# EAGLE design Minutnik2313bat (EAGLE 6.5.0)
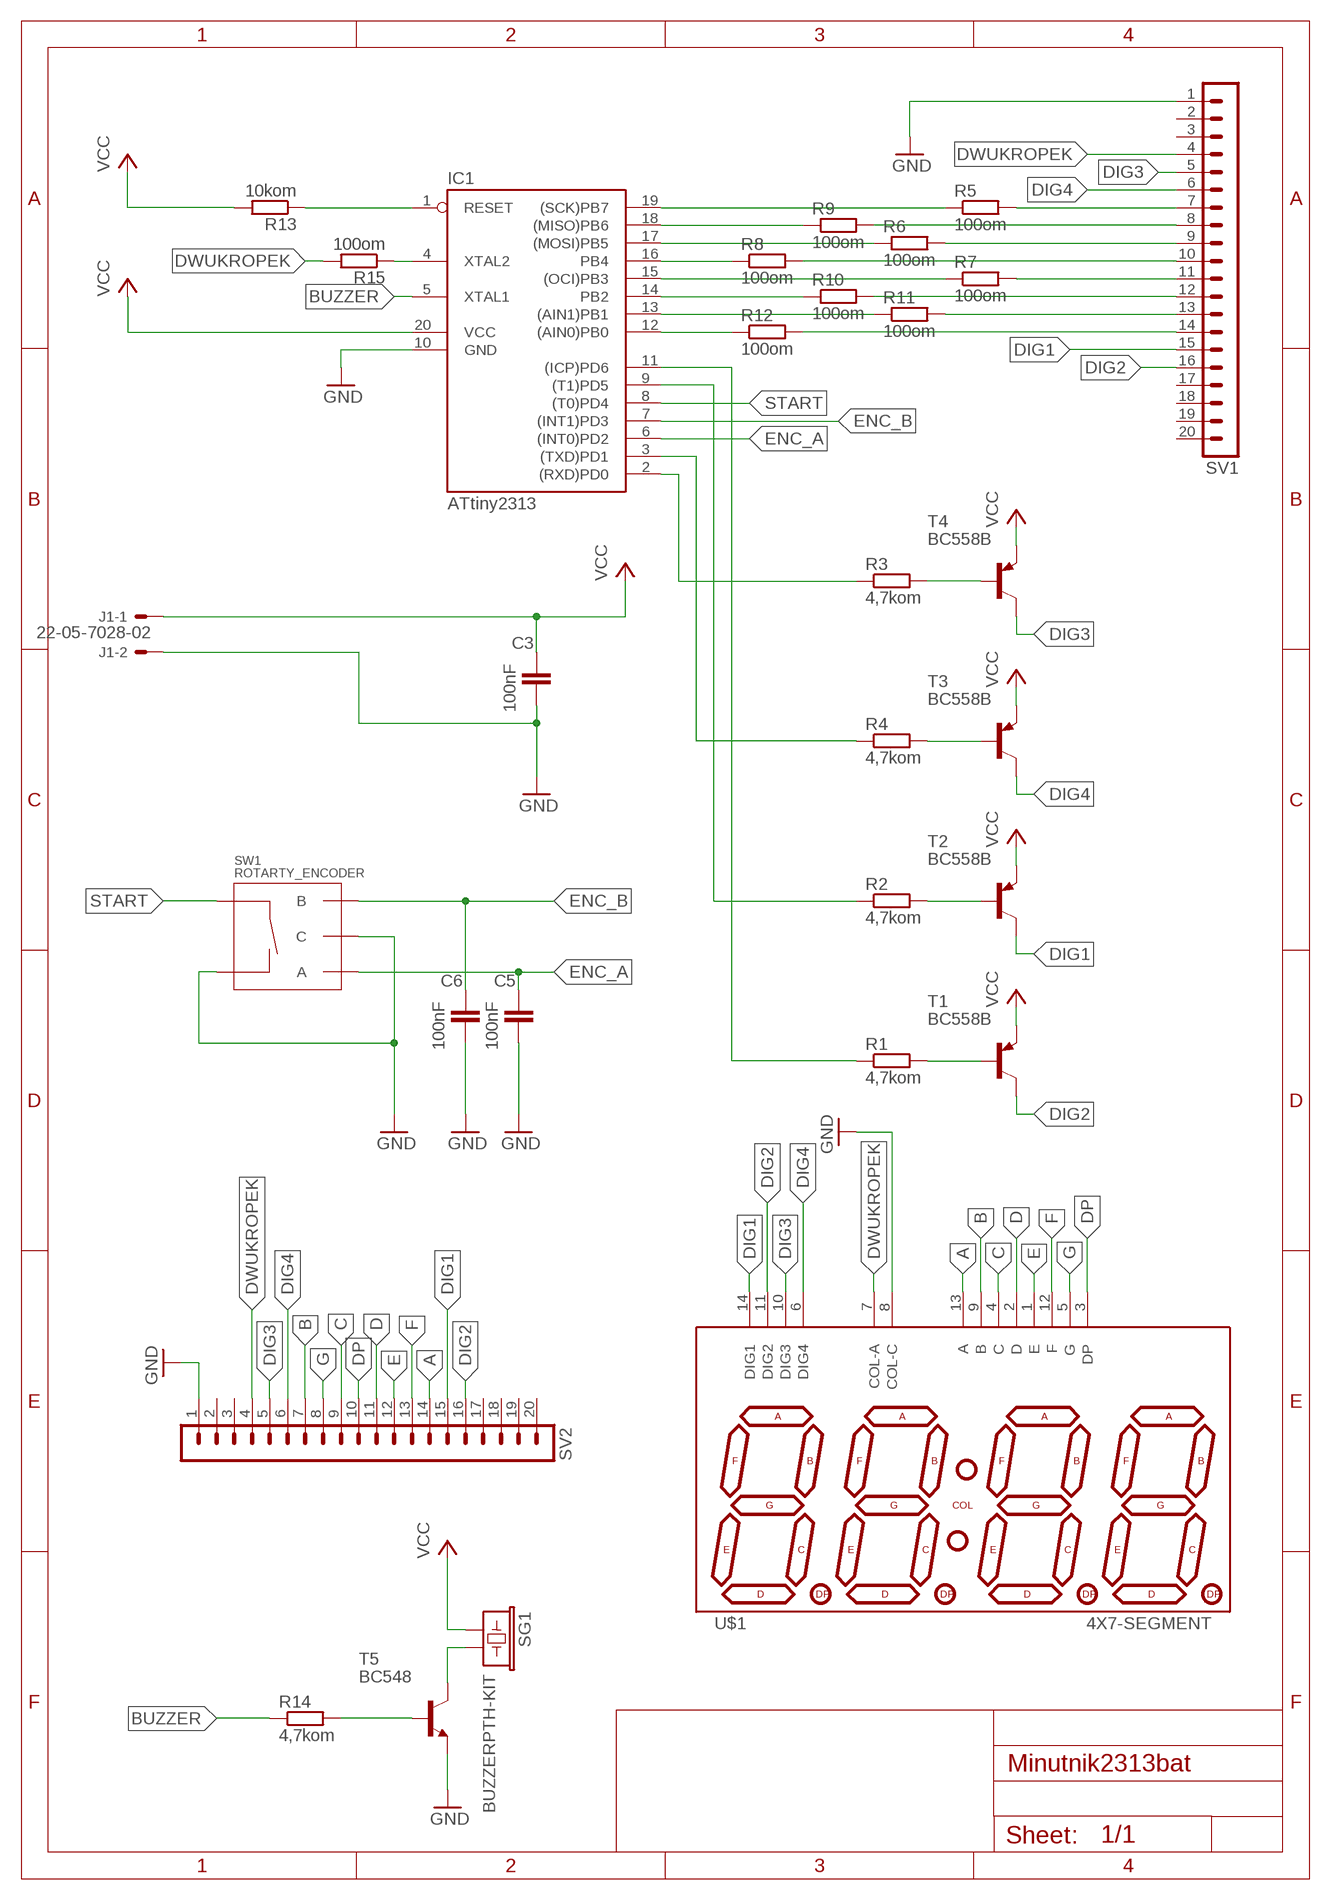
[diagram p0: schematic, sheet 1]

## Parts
C3  100nF  C-EU050-025X075  [C050-025X075]
C5  100nF  C-EU050-025X075  [C050-025X075]
C6  100nF  C-EU050-025X075  [C050-025X075]
IC1  ATtiny2313  AT90S2313P  [DIL20]
J1  22-05-7028-02  [7395-02]
R1  4,7kom  R-EU_0207/7  [0207/7]
R2  4,7kom  R-EU_0207/7  [0207/7]
R3  4,7kom  R-EU_0207/7  [0207/7]
R4  4,7kom  R-EU_0207/7  [0207/7]
R5  100om  R-EU_0207/7  [0207/7]
R6  100om  R-EU_0207/7  [0207/7]
R7  100om  R-EU_0207/7  [0207/7]
R8  100om  R-EU_0207/7  [0207/7]
R9  100om  R-EU_0207/7  [0207/7]
R10  100om  R-EU_0207/7  [0207/7]
R11  100om  R-EU_0207/7  [0207/7]
R12  100om  R-EU_0207/7  [0207/7]
R13  10kom  R-EU_0207/7  [0207/7]
R14  4,7kom  R-EU_0207/7  [0207/7]
R15  100om  R-EU_0207/7  [0207/7]
SG1  BUZZERPTH-KIT  [BUZZER-12MM-KIT]
SV1  MA20-1  [MA20-1]
SV2  MA20-1  [MA20-1]
SW1  ROTARTY_ENCODER  [ROTARY_ENC_PLAIN]
T1  BC558B  [TO92-EBC]
T2  BC558B  [TO92-EBC]
T3  BC558B  [TO92-EBC]
T4  BC558B  [TO92-EBC]
T5  BC548  [TO92-EBC]
U$1  4X7-SEGMENT  [4X7-SEGMENT]

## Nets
A: SV2.14 U$1.13(A)
B: SV2.7 U$1.9(B)
BUZZER: IC1.5(XTAL1) R14.1
C: SV2.9 U$1.4(C)
D: SV2.11 U$1.2(D)
DIG1: SV1.15 SV2.15 T2.C U$1.14(DIG1)
DIG2: SV1.16 SV2.16 T1.C U$1.11(DIG2)
DIG3: SV1.5 SV2.5 T4.C U$1.10(DIG3)
DIG4: SV1.6 SV2.6 T3.C U$1.6(DIG4)
DP: SV2.10 U$1.3(DP)
DWUKROPEK: R15.2 SV1.4 SV2.4 U$1.7(COL-A)
E: SV2.12 U$1.1(E)
ENC_A: C5.1 IC1.6((INT0)PD2) SW1.A
ENC_B: C6.1 IC1.7((INT1)PD3) SW1.B
F: SV2.13 U$1.12(F)
G: SV2.8 U$1.5(G)
GND: C3.2 C5.2 C6.2 IC1.10(GND) J1.2 SV1.1 SV2.1 SW1.C SW1.SW- T5.E U$1.8(COL-C)
N$1: IC1.19((SCK)PB7) R5.1
N$2: IC1.18((MISO)PB6) R9.1
N$3: IC1.17((MOSI)PB5) R6.1
N$4: IC1.16(PB4) R8.1
N$5: IC1.15((OCI)PB3) R7.1
N$6: IC1.14(PB2) R10.1
N$7: IC1.13((AIN1)PB1) R11.1
N$8: IC1.12((AIN0)PB0) R12.1
N$9: R5.2 SV1.7
N$10: R4.2 T3.B
N$11: R3.2 T4.B
N$12: IC1.4(XTAL2) R15.1
N$16: R9.2 SV1.8
N$17: R6.2 SV1.9
N$18: R8.2 SV1.10
N$19: R7.2 SV1.11
N$20: R10.2 SV1.12
N$21: R11.2 SV1.13
N$22: R12.2 SV1.14
N$23: IC1.3((TXD)PD1) R4.1
N$24: IC1.2((RXD)PD0) R3.1
N$25: IC1.1(RESET) R13.1
N$26: IC1.11((ICP)PD6) R1.1
N$27: IC1.9((T1)PD5) R2.1
N$30: R1.2 T1.B
N$31: R2.2 T2.B
N$50: R14.2 T5.B
N$51: SG1.- T5.C
START: IC1.8((T0)PD4) SW1.SW+
VCC: C3.1 IC1.20(VCC) J1.1 R13.2 SG1.+ T1.E T2.E T3.E T4.E
Unconnected: SV1.2 SV1.3 SV1.17 SV1.18 SV1.19 SV1.20 SV2.2 SV2.3 SV2.17 SV2.18 SV2.19 SV2.20

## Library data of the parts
C3 C5 C6 = rcl:C-EU: CAPACITOR, European symbol
IC1 = atmel:AT90S2313: MICROCONTROLLER 2 Kbytes FLASH 128 bytes SRAM 128 bytes EEPROM UART; OC_FARNELL: unknown; OC_NEWARK: unknown
J1 = con-molex:22-?-02: CONNECTOR; OC_FARNELL: 9731601; OC_NEWARK: unknown
R1-R15 = rcl:R-EU_: RESISTOR, European symbol
SG1 = SparkFun-Electromechanical:BUZZER: Buzzer 12mm; PROD_ID: COMP-08253
SV1 SV2 = con-lstb:MA20-1: PIN HEADER; OC_FARNELL: unknown; OC_NEWARK: unknown
SW1 = SparkFun-Electromechanical:ROTARTY_ENCODER: Simple no LED rotary encoder Example: COM-09117
T1-T4 = transistor-pnp:BC558*: PNP Transistror
T5 = transistor-npn:BC548*: NPN Transistor
U$1 = moje:4X7-SEGMENT

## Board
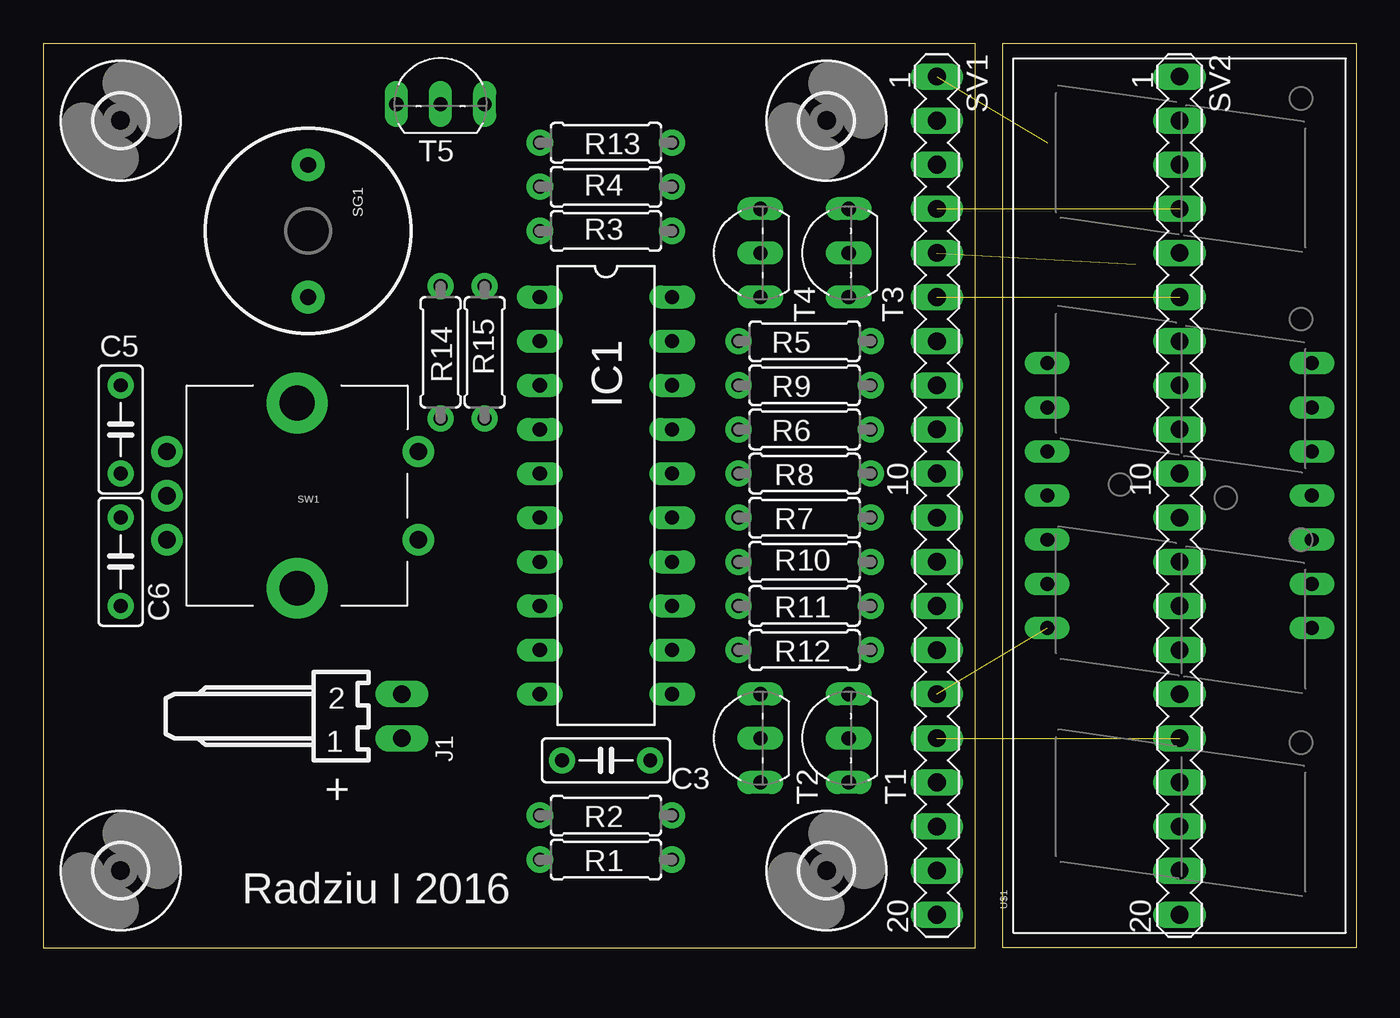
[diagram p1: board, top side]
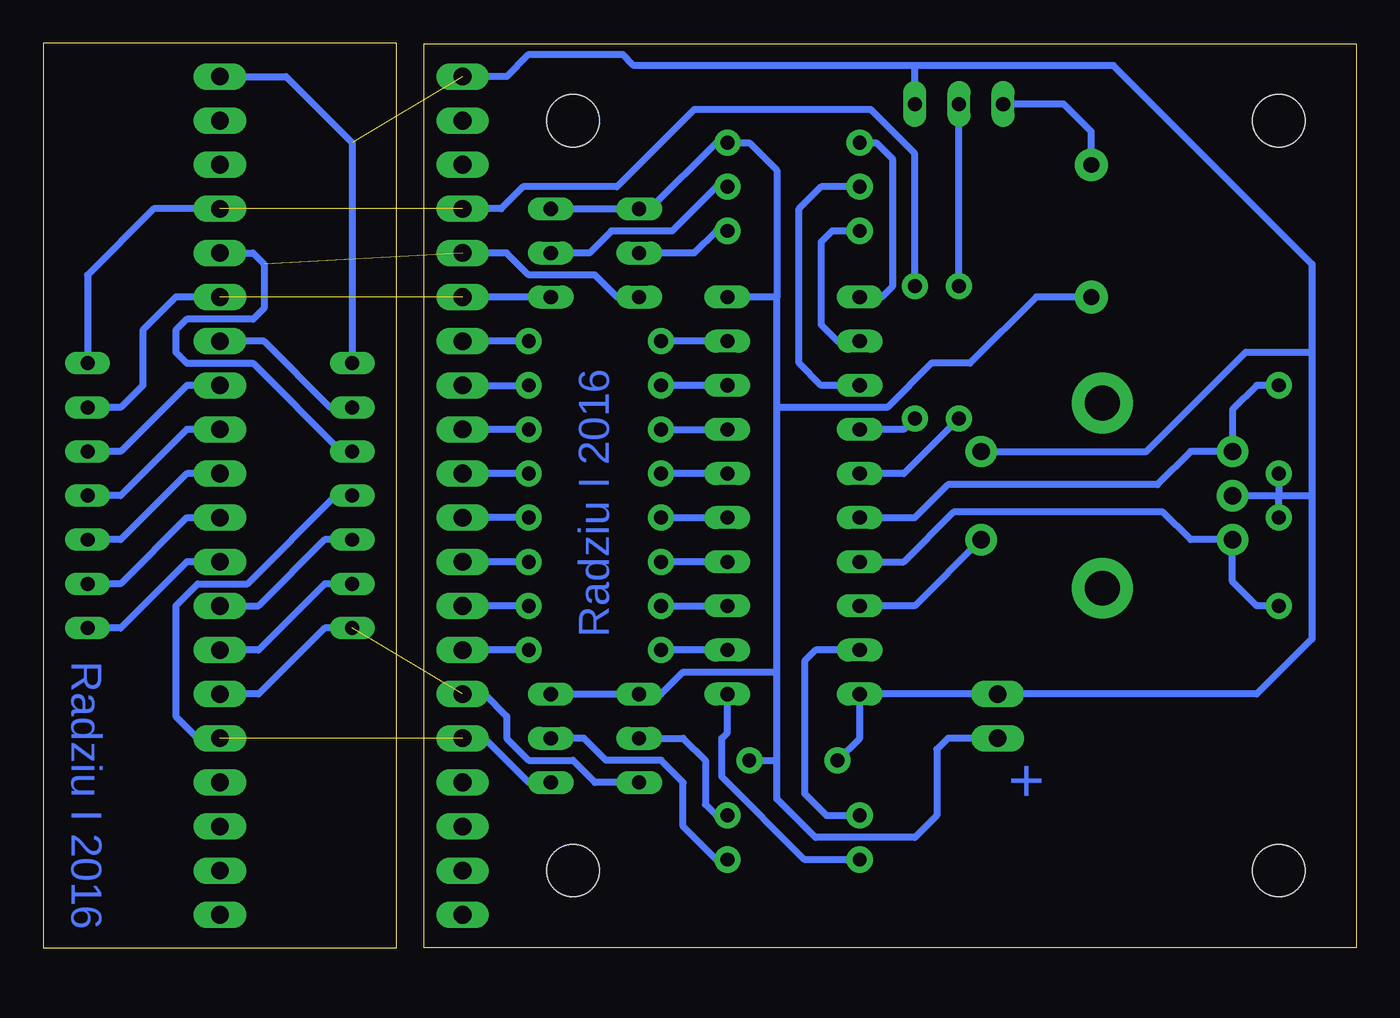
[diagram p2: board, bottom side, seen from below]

Size 75.56 x 52.07 mm. Coordinates in mm from the lower left corner, seen from the top.
Outline: 0,0 53.65,0 53.65,52.06 0,52.06 0,0
Outline: 55.24,0 55.24,52.07 75.56,52.07 75.56,0 55.24,0
Copper layers (1*16): Top 0.035mm / dielectric 1.5mm / Bottom 0.035mm
Design rules "default": minimum track width 10mil, minimum drill 24mil, track to track 8mil, track to pad 8mil, pad to pad 8mil, via to via 8mil, smd to smd 8mil, copper to edge 40mil, drill to drill 8mil, minimum pad ring 10mil, minimum via ring 8mil, stop-mask expansion 4mil, vias tented up to drill 0mil, thermal gap 10mil

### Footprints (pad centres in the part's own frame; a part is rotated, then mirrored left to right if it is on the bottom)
C050-025X075 = drill 0.8 pad 1.5: 1 -2.54,0; 2 2.54,0
DIL20 = drill 0.813 long: 1 -11.43,-3.81; 2 -8.89,-3.81; 3 -6.35,-3.81; 4 -3.81,-3.81; 5 -1.27,-3.81; 6 1.27,-3.81; 7 3.81,-3.81; 8 6.35,-3.81; 9 8.89,-3.81; 10 11.43,-3.81; 11 11.43,3.81; 12 8.89,3.81; 13 6.35,3.81; 14 3.81,3.81; 15 1.27,3.81; 16 -1.27,3.81; 17 -3.81,3.81; 18 -6.35,3.81; 19 -8.89,3.81; 20 -11.43,3.81
7395-02 = drill 1.016 long: 1 1.27,0; 2 -1.27,0
0207/7 = drill 0.8 pad 1.5: 1 -3.81,0; 2 3.81,0
BUZZER-12MM-KIT = drill 0.9 pad 1.88: + 3.809,0; - -3.809,0
MA20-1 = drill 1.016 long: 1 -24.13,0; 2 -21.59,0; 3 -19.05,0; 4 -16.51,0; 5 -13.97,0; 6 -11.43,0; 7 -8.89,0; 8 -6.35,0; 9 -3.81,0; 10 -1.27,0; 11 1.27,0; 12 3.81,0; 13 6.35,0; 14 8.89,0; 15 11.43,0; 16 13.97,0; 17 16.51,0; 18 19.05,0; 19 21.59,0; 20 24.13,0
ROTARY_ENC_PLAIN = drill 1 pad 1.8: A 7.493,-2.54; B 7.493,2.54; C 7.493,0; SW+ -6.985,2.54; SW- -6.985,-2.54 | drill 2 pad 3.5: P$3 0,5.334; P$4 0,-5.334
TO92-EBC = drill 0.813 long: B 0,-1.27; C -2.54,-1.27; E 2.54,-1.27
4X7-SEGMENT = drill 0.8 long: 1 -7.62,-7.62; 2 -5.08,-7.62; 3 -2.54,-7.62; 4 0,-7.62; 5 2.54,-7.62; 6 5.08,-7.62; 7 7.62,-7.62; 8 7.62,7.62; 9 5.08,7.62; 10 2.54,7.62; 11 0,7.62; 12 -2.54,7.62; 13 -5.08,7.62; 14 -7.62,7.62
3,0 = hole 3: 0,0

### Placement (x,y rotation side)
C3  32.39,10.79 180 top
C5  4.45,29.84 270 top
C6  4.45,22.23 90 top
IC1  32.38,26.04 270 top
J1  20.64,13.34 270 top
R1  32.38,5.08 0 top
R2  32.38,7.62 0 top
R3  32.38,41.27 0 top
R4  32.38,43.81 0 top
R5  43.81,34.92 0 top
R6  43.81,29.84 0 top
R7  43.81,24.77 0 top
R8  43.81,27.3 0 top
R9  43.81,32.38 0 top
R10  43.81,22.23 0 top
R11  43.81,19.68 0 top
R12  43.81,17.14 0 top
R13  32.38,46.35 0 top
R14  22.86,34.29 90 top
R15  25.4,34.29 90 top
SG1  15.24,41.27 270 top
SV1  51.44,26.04 270 top
SV2  65.41,26.04 270 top
SW1  14.61,26.04 180 top
T1  45.09,12.06 90 top
T2  40.01,12.06 90 top
T3  45.09,40.01 90 top
T4  40.01,40.01 90 top
T5  22.86,49.85 0 top
U$1  65.41,26.04 90 top
U$2  [3,0]  45.09,4.45 0 top
U$3  [3,0]  45.09,47.62 0 top
U$4  [3,0]  4.45,4.45 0 top
U$5  [3,0]  4.45,47.62 0 top

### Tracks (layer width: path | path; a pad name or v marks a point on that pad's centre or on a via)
A
  Bottom 0.406: U$1.13 59.37,20.95 63.18,17.14 SV2.14
B
  Bottom 0.406: SV2.7 62.87,34.92 59.05,31.11 U$1.9
BUZZER
  Bottom 0.406: R14.1 26.04,27.3 IC1.5
C
  Bottom 0.406: SV2.9 67.31,29.84 71.12,26.04 U$1.4
D
  Bottom 0.406: SV2.11 67.31,24.77 71.12,20.95 U$1.2
DIG1  (1 unrouted)
  Bottom 0.406: SV1.15 50.16,14.61 48.9,13.34 48.9,12.06 47.62,10.79 45.09,10.79 43.81,9.53 T2.C | U$1.14 59.37,18.41 63.18,14.61 SV2.15
DIG2  (1 unrouted)
  Bottom 0.406: SV1.16 50.16,12.06 47.62,9.53 T1.C | SV2.16 66.67,12.06 67.94,13.34 67.94,19.68 66.67,20.95 63.82,20.95 58.74,26.04 U$1.11
DIG3  (1 unrouted)
  Bottom 0.406: SV1.5 48.9,40.01 47.62,38.73 43.81,38.73 42.55,37.47 T4.C | SV2.5 63.5,40.01 62.87,39.37 62.87,36.83 63.5,36.2 67.31,36.2 67.94,35.56 67.94,34.29 67.31,33.66 63.5,33.66 58.42,28.57 U$1.10
DIG4  (1 unrouted)
  Bottom 0.406: SV2.6 67.94,37.47 69.85,35.56 69.85,32.38 71.12,31.11 U$1.6 | T3.C SV1.6
DP
  Bottom 0.406: SV2.10 67.31,27.3 71.12,23.5 U$1.3
DWUKROPEK  (1 unrouted)
  Bottom 0.406: R15.2 25.4,45.72 27.94,48.26 38.1,48.26 42.55,43.81 47.94,43.81 49.21,42.55 SV1.4 | SV2.4 69.22,42.55 73.03,38.73 U$1.7
E
  Bottom 0.406: SV2.12 67.31,22.23 71.12,18.41 U$1.1
ENC_A
  Bottom 0.406: IC1.6 25.4,24.77 23.5,26.67 11.43,26.67 9.53,28.57 SW1.A 7.11,30.99 5.71,32.38 C5.1
ENC_B
  Bottom 0.406: IC1.7 26.04,22.23 23.18,25.08 11.11,25.08 9.53,23.5 SW1.B 7.11,21.08 5.71,19.68 C6.1
F
  Bottom 0.406: SV2.13 63.18,19.68 59.37,23.5 U$1.12
G
  Bottom 0.406: SV2.8 67.31,32.38 71.12,28.57 U$1.5
GND  (1 unrouted)
  Bottom 0.406: SV2.1 61.59,50.16 57.78,46.35 U$1.8 | SV1.1 48.9,50.16 47.62,51.44 42.23,51.44 41.59,50.8 25.4,50.8 | 25.4,50.8 13.97,50.8 2.54,39.37 2.54,34.29 | T5.E 25.4,50.8 | 2.54,34.29 2.54,26.04 | 2.54,26.04 2.54,17.78 5.71,14.61 J1.2 IC1.10 28.57,12.07 C3.2 | SW1.SW- 12.06,28.57 6.35,34.29 2.54,34.29 | SW1.C 4.45,26.04 | 4.45,26.04 2.54,26.04 | C5.2 4.45,26.04 | C6.2 4.45,26.04
N$1
  Bottom 0.406: IC1.19 R5.1
N$2
  Bottom 0.406: IC1.18 R9.1
N$3
  Bottom 0.406: R6.1 IC1.17
N$4
  Bottom 0.406: IC1.16 R8.1
N$5
  Bottom 0.406: R7.1 IC1.15
N$6
  Bottom 0.406: IC1.14 R10.1
N$7
  Bottom 0.406: R11.1 IC1.13
N$8
  Bottom 0.406: IC1.12 R12.1
N$9
  Bottom 0.406: R5.2 SV1.7
N$10
  Bottom 0.406: T3.B 44.13,40.01 42.86,41.27 39.37,41.27 36.83,43.81 R4.2
N$11
  Bottom 0.406: R3.2 36.83,41.27 38.1,40.01 T4.B
N$12
  Bottom 0.406: R15.1 26.04,29.84 IC1.4
N$16
  Bottom 0.406: SV1.8 R9.2
N$17
  Bottom 0.406: R6.2 SV1.9
N$18
  Bottom 0.406: R8.2 SV1.10
N$19
  Bottom 0.406: R7.2 SV1.11
N$20
  Bottom 0.406: R10.2 SV1.12
N$21
  Bottom 0.406: R11.2 SV1.13
N$22
  Bottom 0.406: R12.2 SV1.14
N$23
  Bottom 0.406: IC1.3 30.8,32.38 32.07,33.66 32.07,42.55 30.8,43.81 R4.1
N$24
  Bottom 0.406: R3.1 30.16,41.27 30.8,40.64 30.8,35.88 29.84,34.92 IC1.2
N$25
  Bottom 0.406: R13.1 27.62,46.35 26.67,45.4 26.67,38.1 27.3,37.47 IC1.1
N$26
  Bottom 0.406: R1.1 31.75,5.08 36.51,9.84 36.51,12.06 36.2,12.38 IC1.11
N$27
  Bottom 0.406: IC1.9 31.11,17.14 31.75,16.51 31.75,8.89 30.48,7.62 R2.1
N$30
  Bottom 0.406: R1.2 36.83,5.08 38.73,6.99 38.73,9.53 40.01,10.79 43.18,10.79 44.45,12.06 T1.B
N$31
  Bottom 0.406: T2.B 38.73,12.06 37.47,10.79 37.47,8.26 36.83,7.62 R2.2
N$50
  Bottom 0.406: R14.2 T5.B
N$51
  Bottom 0.406: SG1.- 15.24,46.99 16.83,48.58 T5.C
START
  Bottom 0.406: SW1.SW+ 25.4,19.68 IC1.8
VCC
  Bottom 0.406: T1.E T2.E 40.01,14.61 38.73,15.88 33.34,15.88 | 33.34,15.88 33.34,31.11 | 33.34,31.11 33.34,37.47 | 33.34,37.47 IC1.20 | T3.E T4.E 40.64,42.55 36.83,46.35 R13.2 34.92,46.35 33.34,44.77 33.34,37.47 | 33.34,31.11 26.99,31.11 24.45,33.66 22.23,33.66 18.41,37.47 SG1.+ | 33.34,10.79 33.34,8.57 31.11,6.35 25.4,6.35 24.13,7.62 24.13,11.43 23.5,12.06 J1.1 | 33.34,10.79 33.34,15.88 | C3.1 33.34,10.79

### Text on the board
Bottom: Radziu I 2016 | Radziu I 2016 | +
tPlace: + | Radziu I 2016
